VAR_GLOBAL CONSTANT	
	
	cOversamples			: UDINT := 10;					// number of oversamples
	cSampleRate				: UDINT := 10000;   			// 1ms task with 10 oversamples = 10kHz
	
	// define FFT parameters, note that cFSample / cWindowLength must be such that numerical frequency resolution is lower than fLowerFrequencyLimit
	// resolution  =  10000/4000 = 2.5 Hz < 10 Hz 
	cFFTLength				: UDINT	:= 4096;	        			// length of FFT
    cWindowLength			: UDINT := 4000;            			// 96 samples Zero padding
	cWindowType				: E_CM_WindowType := E_CM_WindowType.eCM_HannWindow;
	cOverlap				: UDINT := cWindowLength/2;				// use recommended overlap for applied signal window
	cBufferLength			: UDINT := cWindowLength - cOverlap;	// buffer size due to 50% overlap
	
	// define frequency interval according to ISO 10816-3, e.g. 10 .. 1000 Hz for rotating speed over 600r/min
	cfLowerFrequencyLimit	: UDINT := 10;   
	cfUpperFrequencyLimit	: UDINT := 1000; 
	
	// Parameters for RMS calculation
	cOrderRMS        		: UDINT := 2; 				// ISO 10816-3 requires velocity and displacement, if measured using accelerometer we need to integrate 2 times.
	cChannels		 		: UDINT := 2; 				// ISO 10816-3 says 2 orthogonal sensors per measurement location, i.e. 2 channels.
	
	// Samples to use to calculate mean and empirical standard deviation of RMS values
	cAppendData				: UDINT := 100;				// Number of (integrated) RMS values used for statistical analysis
	cResetData				: BOOL := TRUE;				// Reset internal buffers after calculation in statisticss
	
	// Classes according to ISO: machine type 1, stiff location, Class definitions
	cMaxClasses				: UDINT := 3;
	cISOClassDef_Acc		: ARRAY[1..3] OF LREAL := [1e6, 1e6, 1e6]; 				// in ISO 10816-3 not necessary (but e.g. in -21 for wind turbines)
	cISOClassDef_Vel		: ARRAY[1..3] OF LREAL := [2.3E-3, 4.5E-3, 7.1E-3];
	cISOClassDef_Displ		: ARRAY[1..3] OF LREAL := [29E-6, 57E-6, 90E-6];	
	
	// optional constants if real sensors are applied
	cGravitationalAcc 		: LREAL := 9.81;    // 1 g approx 9.81 m/s^2 -> physical constant
	cSensitivity      		: LREAL := 0.01;    // depends on sensor used in application, e.g. 10 mV/g
	cMeasurementRange 		: LREAL := 5;       // +-5 Volts (EL3632)
	cResolution       		: LREAL := 32768;   // 2^15 (15 bits resolution + 1 bit sign) (EL3632)
	cScale            		: LREAL := cMeasurementRange*cGravitationalAcc/(cSensitivity*cResolution);
	
END_VAR
